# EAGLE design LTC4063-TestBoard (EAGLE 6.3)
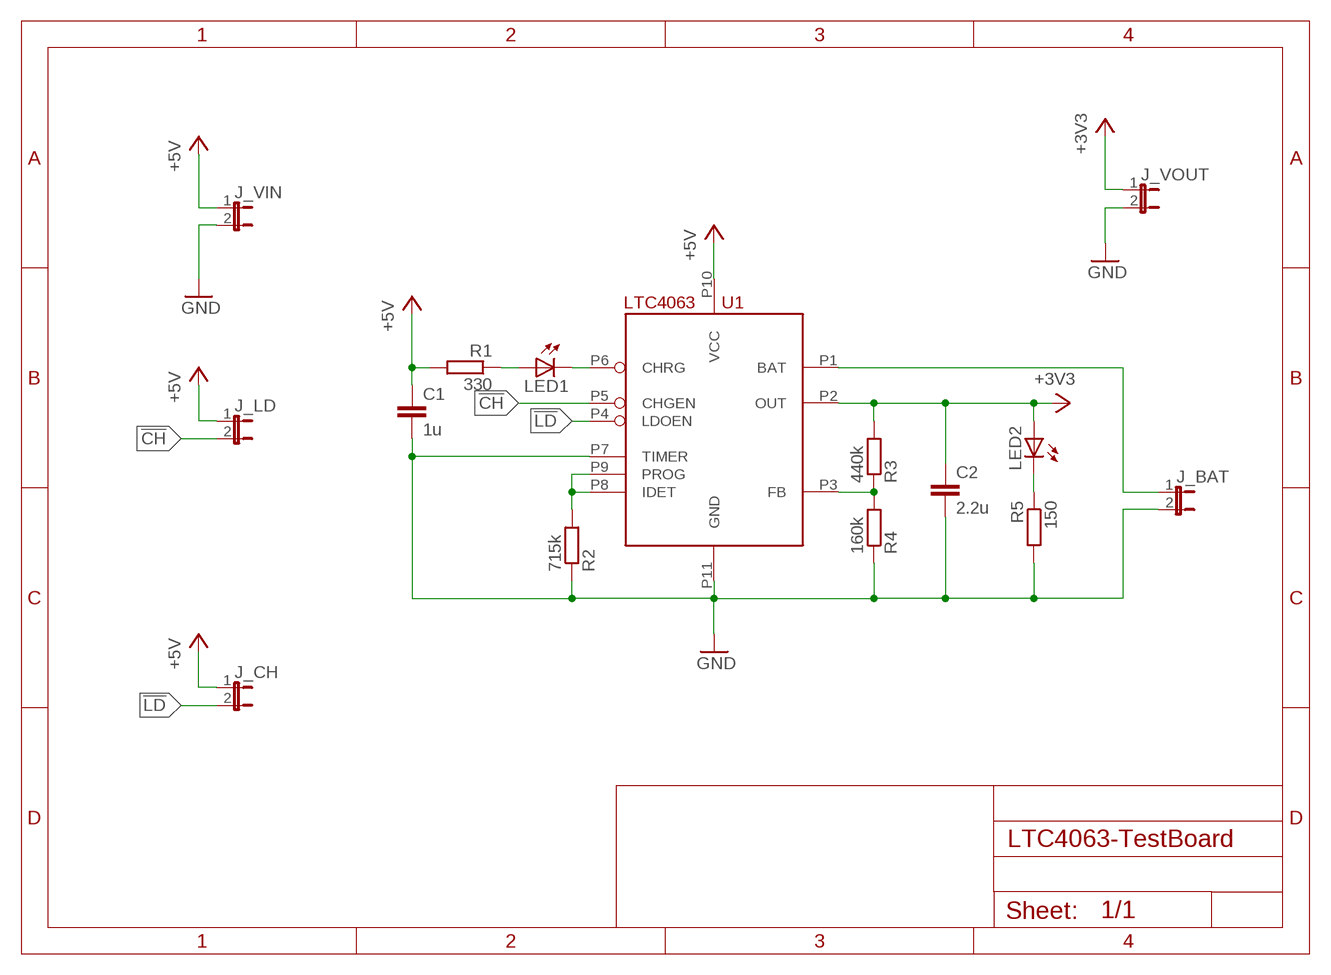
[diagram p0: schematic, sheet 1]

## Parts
C1  1u  C-EUC0805K  [C0805K]
C2  2.2u  C-EUC0805K  [C0805K]
J_BAT  JP1E  [JP1]
J_CH  JP1E  [JP1]
J_LD  JP1E  [JP1]
J_VIN  JP1E  [JP1]
J_VOUT  JP1E  [JP1]
LED1  LED3MM  [LED3MM]
LED2  LED3MM  [LED3MM]
R1  330  R-EU_R0805  [R0805]
R2  715k  R-EU_R0805  [R0805]
R3  440k  R-EU_R0805  [R0805]
R4  160k  R-EU_R0805  [R0805]
R5  150  R-EU_R0805  [R0805]
U1  LTC4063  [LTC4063]

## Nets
!CH: J_LD.2 U1.P5(CHGEN)
!LD: J_CH.2 U1.P4(LDOEN)
+3V3: C2.1 J_VOUT.1 LED2.A R3.2 U1.P2(OUT)
+5V: C1.1 J_CH.1 J_LD.1 J_VIN.1 R1.2 U1.P10(VCC)
GND: C1.2 C2.2 J_BAT.2 J_VIN.2 J_VOUT.2 R2.1 R4.1 R5.2 U1.P7(TIMER) U1.P11(GND)
N$1: R3.1 R4.2 U1.P3(FB)
N$2: J_BAT.1 U1.P1(BAT)
N$3: LED1.K(C) U1.P6(CHRG)
N$4: LED1.A R1.1
N$5: R2.2 U1.P8(IDET) U1.P9(PROG)
N$6: LED2.K(C) R5.1

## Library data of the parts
C1 C2 = rcl:C-EU: CAPACITOR, European symbol
J_BAT J_CH J_LD J_VIN J_VOUT = jumper:JP1E: JUMPER
LED1 LED2 = led:LED: LED
R1-R5 = rcl:R-EU_: RESISTOR, European symbol
U1 = LinearTechnology:LTC4063: LTC4063 - Standalone Linear Li-Ion Charger with Micropower Low Dropout Linear Regulator The LTC®4063 is a standalone linear charger for single cell lithium-ion batteries with an adjustable low dropout linear regulator (LDO). The adjustable LDO regulates an output voltage between 1.2V to 4.2V at up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

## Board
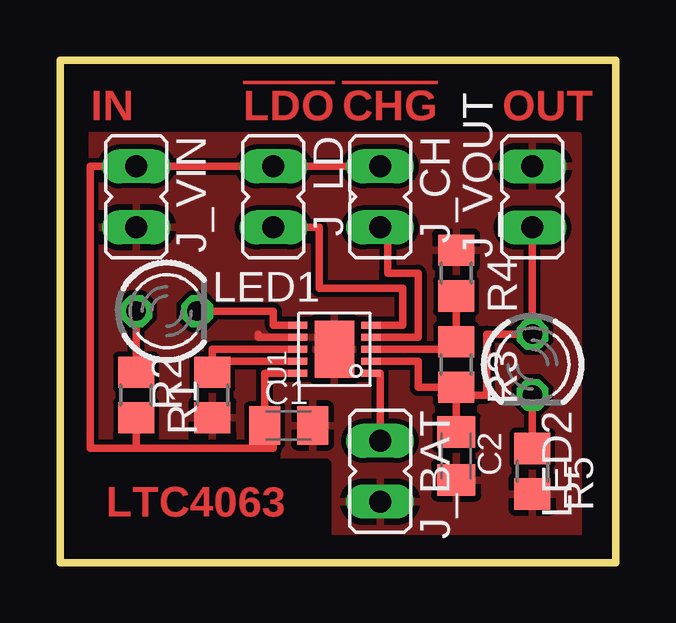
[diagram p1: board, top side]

Size 23.16 x 20.95 mm. Coordinates in mm from the lower left corner, seen from the top.
Outline: 0,0 23.16,0 23.16,20.95 0,20.95 0,0
Copper layers (1*16): Top 0.035mm / dielectric 1.5mm / Bottom 0.035mm
Design rules "default": minimum track width 10mil, minimum drill 24mil, track to track 8mil, track to pad 8mil, pad to pad 8mil, via to via 8mil, smd to smd 8mil, copper to edge 40mil, drill to drill 8mil, minimum pad ring 10mil, minimum via ring 8mil, stop-mask expansion 4mil, vias tented up to drill 0mil, thermal gap 10mil
tRestrict: area 1,1 to 11.1,4.1

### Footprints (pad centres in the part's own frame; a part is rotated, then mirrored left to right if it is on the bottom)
C0805K = smd 1.3 x 1.6: 1 -1,0; 2 1,0
JP1 = drill 0.914 long: 1 0,-1.27; 2 0,1.27
LED3MM = drill 0.813 octagon: A -1.27,0; K 1.27,0
R0805 = smd 1.3 x 1.5: 1 -0.95,0; 2 0.95,0
LTC4063 = smd 0.3 x 0.8: P1 -1,-1.525; P2 -0.5,-1.525; P3 0,-1.525; P4 0.5,-1.525; P5 1,-1.525; P6 1,1.525; P7 0.5,1.525; P8 0,1.525; P9 -0.5,1.525; P10 -1,1.525 | smd 2.38 x 1.65: P11 0,0

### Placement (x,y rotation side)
C1  9.53,5.71 0 top
C2  16.51,4.45 270 top
J_BAT  13.34,3.81 180 top
J_CH  13.34,15.24 180 top
J_LD  8.89,15.24 180 top
J_VIN  3.17,15.24 180 top
J_VOUT  19.68,15.24 0 top
LED1  4.45,10.48 0 top
LED2  19.68,8.26 270 top
R1  3.17,6.99 270 top
R2  6.35,6.99 90 top
R3  16.51,8.26 270 top
R4  16.51,12.06 270 top
R5  19.68,3.81 270 top
U1  11.43,8.89 90 top

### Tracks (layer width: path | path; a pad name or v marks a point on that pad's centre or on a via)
!CH
  Top 0.305: J_LD.2 10.79,13.97 10.79,13.34 10.79,11.43 14.29,11.43 14.29,9.89 U1.P5
!LD
  Top 0.305: J_CH.2 13.65,13.97 13.65,13.34 13.65,12.06 14.92,12.06 14.92,9.39 U1.P4
+3V3
  Top 0.305: U1.P2 14.92,8.39 14.92,7.3 R3.2 | R3.2 C2.1 | R3.2 15.88,6.99 17.78,6.99 17.78,9.53 LED2.A J_VOUT.1
+5V
  Top 0.305: U1.P10 8.53,7.89 C1.1 8.89,5.71 8.89,4.76 3.17,4.76 R1.2 3.17,4.76 1.27,4.76 1.27,16.51 J_VIN.1 J_LD.1 J_CH.1
GND
  Top 0.305: U1.P7 8.26,9.39 8.26,9.53
  pour Top: 0,17.78 0,0 21.59,0 21.59,17.78
N$1
  Top 0.305: U1.P3 15.88,8.89 R3.1 R4.2
N$2
  Top 0.305: J_BAT.1 13.34,7.89 U1.P1
N$3
  Top 0.305: U1.P6 8.89,9.89 8.89,10.48 LED1.K
N$4
  Top 0.305: R1.1 LED1.A
N$5
  Top 0.305: U1.P9 6.35,8.39 R2.2 6.35,8.89 U1.P8
N$6
  Top 0.305: LED2.K R5.1

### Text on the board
Top: IN | !LDO | !CHG | OUT | LTC4063

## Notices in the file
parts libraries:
LinearTechnology: Copyright (c) 2013, Michael Hohl
